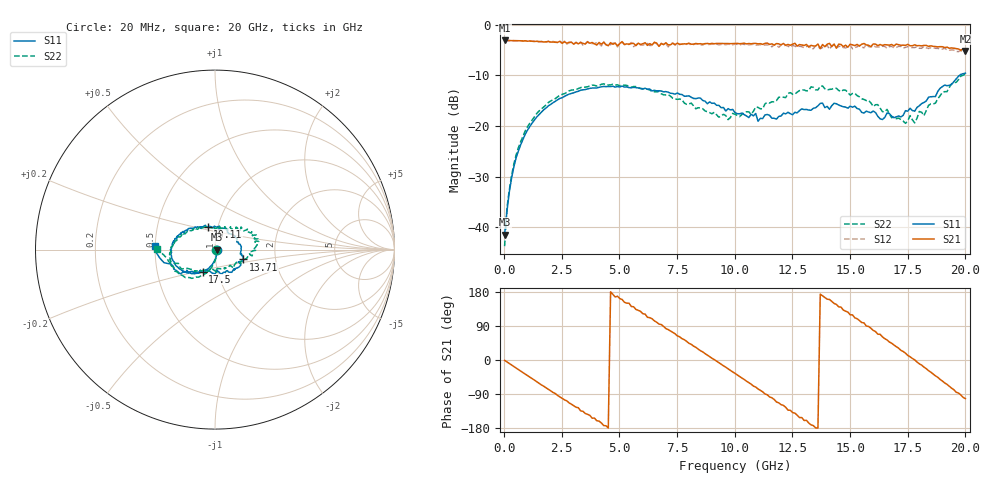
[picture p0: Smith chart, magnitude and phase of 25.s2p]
!Agilent Technologies,N5230A,US43500223,A.07.50.48
!Agilent N5230A: A.07.50.48
!Date: Tuesday, September 15, 2015 13:09:42
!Correction: S11(Full 2 Port(1,2))
!S21(Full 2 Port(1,2))
!S12(Full 2 Port(1,2))
!S22(Full 2 Port(1,2))
!S2P File: Measurements: S11, S21, S12, S22:
# Hz S  dB  R 50
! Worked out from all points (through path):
!   201 points, 20 MHz to 20 GHz, reference 50 ohm
!   highest |S21| = -3.09 dB at 20 MHz (marker M1); lowest = -5.2 dB at 20 GHz (marker M2)
!   group delay of S21, straight-line fit = 113 ps
!   lowest |S11| = -41.5 dB at 20 MHz (marker M3), VSWR 1.02, Z = 50.8 - j0.0845 ohm
!   |S11| at or under -10 dB: start of sweep to 19.74 GHz
!   |S22| runs from -43.8 to -9.8 dB; largest |S21 - S12| = 0.097
!   S11 on the Smith chart (normalised r, x): 20 MHz: 1.02, -0.00; 10.11 GHz: 0.89, +0.23; 13.71 GHz: 1.37, -0.15; 17.5 GHz: 0.85, -0.21; 20 GHz: 0.50, +0.02
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2e7  -41.46 -5.6  -3.09 -0.9  -3.09 -0.9  -43.76 -11.4
1.199e8  -36.92 -48.7  -3.11 -5.0  -3.10 -5.1  -36.31 -49.2
3.197e8  -30.37 -73.9  -3.12 -13.2  -3.12 -13.3  -29.87 -75.2
9.191e8  -21.57 -100.2  -3.16 -37.4  -3.18 -37.7  -20.91 -98.3
2.1179e9  -15.39 -128.8  -3.39 -85.6  -3.27 -85.5  -14.80 -122.3
3.4166e9  -12.84 -153.5  -3.66 -135.4  -4.02 -137.1  -12.27 -144.3
4.3157e9  -12.18 -168.9  -3.46 -173.0  -3.32 -171.1  -11.67 -160.5
5.1149e9  -12.09 180.0  -3.31 159.7  -3.45 157.6  -11.87 -174.4
6.7133e9  -13.03 160.0  -4.25 94.8  -4.25 92.7  -13.16 161.3
7.3127e9  -13.57 156.0  -3.63 72.8  -3.63 70.5  -14.52 151.9
8.4116e9  -14.47 143.6  -3.76 28.7  -3.74 25.2  -16.38 125.7
1.001e10  -17.35 111.5  -3.68 -35.3  -3.79 -38.4  -17.69 77.5
1.01099e10  -17.57 108.0  -3.67 -39.5  -3.86 -42.8  -17.92 79.8
1.16084e10  -18.45 55.3  -3.75 -99.7  -4.35 -103.3  -15.21 45.3
1.34066e10  -16.51 -9.1  -4.18 -173.1  -4.71 -174.8  -12.35 18.3
1.37063e10  -15.53 -19.1  -4.68 173.8  -4.73 169.7  -12.13 14.0
1.46054e10  -16.04 -40.1  -3.87 139.7  -4.15 135.2  -13.21 1.5
1.55045e10  -17.31 -59.5  -3.83 98.9  -4.41 95.6  -14.61 -12.7
1.67033e10  -17.55 -96.1  -4.03 47.4  -4.29 46.2  -17.63 -45.8
1.75025e10  -17.06 -119.3  -3.86 12.1  -4.31 10.2  -18.98 -86.1
1.91009e10  -11.91 -154.9  -4.49 -60.6  -4.62 -64.4  -13.21 -153.0
2e10  -9.54 176.8  -5.18 -101.8  -5.56 -107.7  -9.77 179.0
